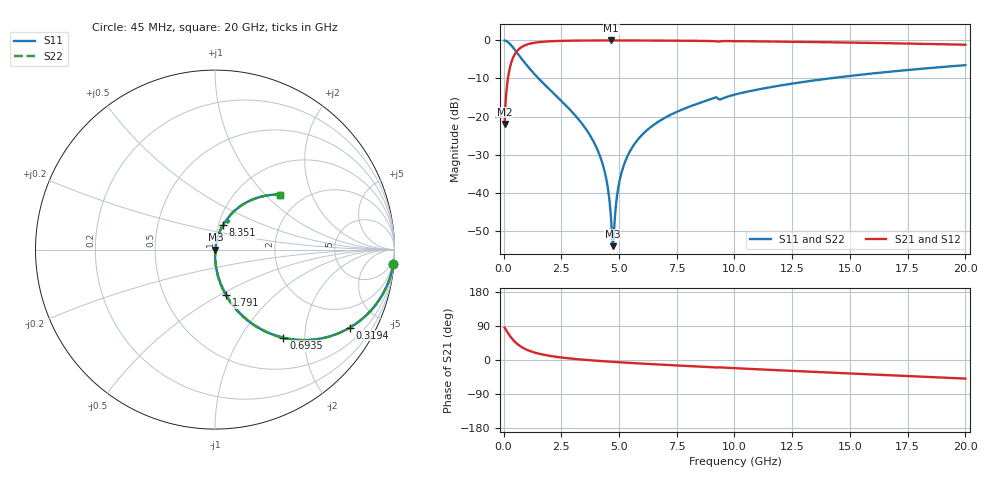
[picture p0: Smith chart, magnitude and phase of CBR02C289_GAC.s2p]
! S-parameter model data by Modelithics Inc.  support@modelithics.com 813-866-6335  Tampa FL USA
! S-Parameter data specifications:
! Substrate: 20-mil Rogers 4350B, substrate thickness, H=0.508mm, Dielectric constant, Er=3.75
! PCB Mounting Pad Footprint: Pad width, PadW=0.32mm , Pad length, PadL=0.37mm , Pad gap, PadG (edge-to-edge)=0.19mm , Reference planes=0.93mm apart
#  GHz  S  MA  R 50
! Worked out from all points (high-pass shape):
!   801 points, 45 MHz to 20 GHz, reference 50 ohm
!   highest |S21| = -0.02 dB at 4.66 GHz (marker M1); lowest = -22.0 dB at 45 MHz (marker M2)
!   |S21| within 3 dB of the highest: 555.6 MHz to end of sweep
!   lowest |S11| = -54.1 dB at 4.734 GHz (marker M3), VSWR 1.00, Z = 50.2 - j0.0225 ohm
!   |S11| at or under -10 dB: 1.516 GHz to 14.1 GHz (12.59 GHz wide, 161 % of centre)
!   |S22| runs from -54.1 to 0.0 dB; largest |S21 - S12| = 0
!   S11 on the Smith chart (normalised r, x): 45 MHz: 1, -25; 319.4 MHz: 0.98, -3.48; 693.5 MHz: 0.98, -1.57; 1.791 GHz: 0.99, -0.53; 8.351 GHz: 1.05, +0.30; 20 GHz: 1.54, +1.22
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0.045  0.9968 -4.6  0.07963 85.4  0.07963 85.4  0.9968 -4.6
0.194662  0.9449 -19.3  0.3271 70.7  0.3271 70.7  0.9449 -19.3
0.319381  0.8688 -30.0  0.4948 60.0  0.4948 60.0  0.8688 -30.0
0.693538  0.6219 -52.2  0.7822 37.7  0.7822 37.7  0.6219 -52.2
1.142525  0.4209 -66.1  0.9059 23.7  0.9059 23.7  0.4209 -66.1
1.791063  0.2602 -76.5  0.9641 13.2  0.9641 13.2  0.2602 -76.5
3.387462  0.0812 -87.6  0.9949 1.1  0.9949 1.1  0.0812 -87.6
3.911281  0.04597 -89.1  0.997 -1.4  0.997 -1.4  0.04597 -89.1
4.285437  0.024 -88.5  0.9977 -3.1  0.9977 -3.1  0.024 -88.5
4.509931  0.01185 -84.6  0.9979 -4.0  0.9979 -4.0  0.01185 -84.6
4.659594  0.004343 -67.7  0.9979 -4.6  0.9979 -4.6  0.004343 -67.7
4.734425  0.001981 -6.5  0.9979 -4.9  0.9979 -4.9  0.001981 -6.5
4.809256  0.004207 56.5  0.9979 -5.2  0.9979 -5.2  0.004207 56.5
5.008806  0.01362 75.5  0.9978 -6.0  0.9978 -6.0  0.01362 75.5
5.308131  0.02755 78.6  0.9975 -7.1  0.9975 -7.1  0.02755 78.6
5.856894  0.05155 78.6  0.9964 -9.0  0.9964 -9.0  0.05155 78.6
6.704981  0.08556 76.6  0.9939 -11.9  0.9939 -11.9  0.08556 76.6
8.351269  0.1455 71.9  0.9865 -17.0  0.9865 -17.0  0.1455 71.9
10.0225  0.1945 67.4  0.9775 -21.6  0.9775 -21.6  0.1945 67.4
13.36496  0.2954 58.3  0.952 -31.1  0.952 -31.1  0.2954 58.3
16.68248  0.3866 49.4  0.9184 -40.1  0.9184 -40.1  0.3866 49.4
20  0.4728 40.5  0.8768 -49.1  0.8768 -49.1  0.4728 40.5
